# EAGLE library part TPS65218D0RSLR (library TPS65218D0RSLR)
Power Management Specialised - PMIC Source: Datasheet
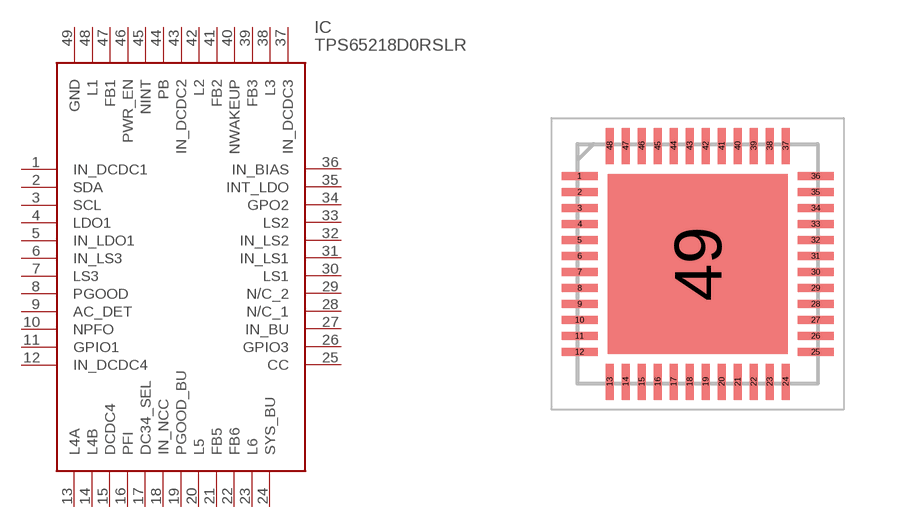
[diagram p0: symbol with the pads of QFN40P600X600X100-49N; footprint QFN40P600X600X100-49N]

Designator prefix IC

## TPS65218D0RSLR (Description: Power Management Specialised - PMIC; Height: 1mm; Manufacturer_Name: Texas Instruments; Manufacturer_Part_Number: TPS65218D0RSLR; Mouser_Part_Number: 595-TPS65218D0RSLR; Mouser_Price-Stock: https://www.mouser.co.uk/ProductDetail/Texas-Instruments/TPS65218D0RSLR?qs=W0yvOO0ixfG7LzI3qsPe0Q%3D%3D)  [QFN40P600X600X100-49N]
1  IN_DCDC1
2  SDA
3  SCL
4  LDO1
5  IN_LDO1
6  IN_LS3
7  LS3
8  PGOOD
9  AC_DET
10  NPFO
11  GPIO1
12  IN_DCDC4
13  L4A
14  L4B
15  DCDC4
16  PFI
17  DC34_SEL
18  IN_NCC
19  PGOOD_BU
20  L5
21  FB5
22  FB6
23  L6
24  SYS_BU
25  CC
26  GPIO3
27  IN_BU
28  N/C_1
29  N/C_2
30  LS1
31  IN_LS1
32  IN_LS2
33  LS2
34  GPO2
35  INT_LDO
36  IN_BIAS
37  IN_DCDC3
38  L3
39  FB3
40  NWAKEUP
41  FB2
42  L2
43  IN_DCDC2
44  PB
45  NINT
46  PWR_EN
47  FB1
48  L1
49  GND

## Footprint QFN40P600X600X100-49N (pad centres in mm)
RSL (S-PVQFN-N48)
smd 0.9 x 0.2: 1 -2.95,2.2; 2 -2.95,1.8; 3 -2.95,1.4; 4 -2.95,1; 5 -2.95,0.6; 6 -2.95,0.2; 7 -2.95,-0.2; 8 -2.95,-0.6; 9 -2.95,-1; 10 -2.95,-1.4; 11 -2.95,-1.8; 12 -2.95,-2.2; 25 2.95,-2.2; 26 2.95,-1.8; 27 2.95,-1.4; 28 2.95,-1; 29 2.95,-0.6; 30 2.95,-0.2; 31 2.95,0.2; 32 2.95,0.6; 33 2.95,1; 34 2.95,1.4; 35 2.95,1.8; 36 2.95,2.2
smd 0.2 x 0.9: 13 -2.2,-2.95; 14 -1.8,-2.95; 15 -1.4,-2.95; 16 -1,-2.95; 17 -0.6,-2.95; 18 -0.2,-2.95; 19 0.2,-2.95; 20 0.6,-2.95; 21 1,-2.95; 22 1.4,-2.95; 23 1.8,-2.95; 24 2.2,-2.95; 37 2.2,2.95; 38 1.8,2.95; 39 1.4,2.95; 40 1,2.95; 41 0.6,2.95; 42 0.2,2.95; 43 -0.2,2.95; 44 -0.6,2.95; 45 -1,2.95; 46 -1.4,2.95; 47 -1.8,2.95; 48 -2.2,2.95
smd 4.5 x 4.5: 49 0,0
